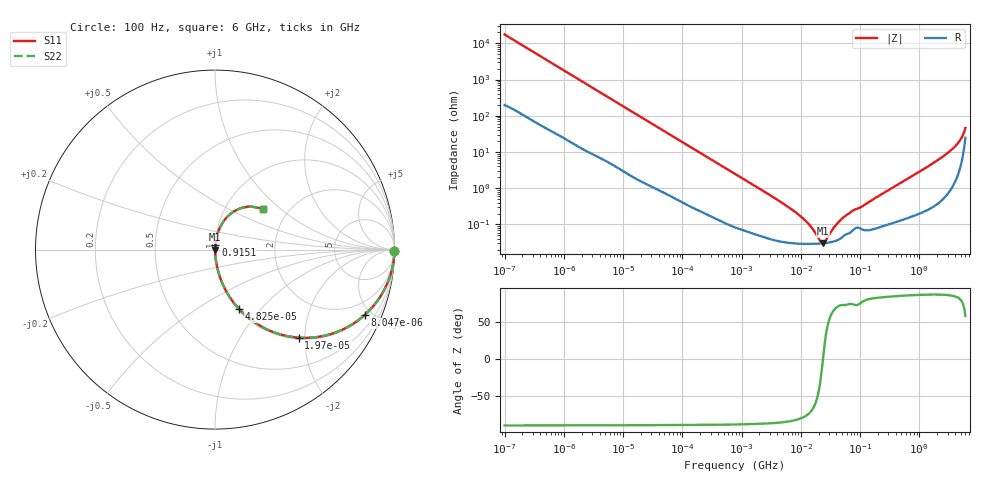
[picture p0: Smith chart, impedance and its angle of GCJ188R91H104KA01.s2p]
!Murata Part Number: GCJ188R91H104KA01
!These Parameters are Measured in Series Mode Connection
!Data Generated on Mar 13, 2026
!  o--ll--o
!Port1  Port2
!  o------o
!Operation Temp=25[degC], DC Bias Voltage=0[V]
!Freq. Start=100[Hz] Stop=6[GHz] 401[Steps]
# Hz S RI R 50
!Freq.(Hz) S11(Real) S11(Imag) S21(Real) S21(Imag) S12(Real) S12(Imag) S22(Real) S22(Imag)
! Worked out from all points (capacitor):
!   401 points, 100 Hz to 6 GHz, reference 50 ohm
!   read as one part in series: C = 90.4 nF near 109 Hz
!   lowest |Z| = 30.3 mohm at 23.28 MHz (marker M1)
!   series resonance near 23.65 MHz, so ESL is about 500 pH
!   S11 on the Smith chart (normalised r, x): 100 Hz: open; 8.047 kHz: 1.07, -4.53; 19.7 kHz: 1.03, -1.87; 48.25 kHz: 1.02, -0.77; 915.1 MHz: 1.00, +0.05; 6 GHz: 1.50, +0.78
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100  0.9999 -0.0057  9.63e-05 0.0057  9.63e-05 0.0057  0.9999 -0.0057
2008  0.9862 -0.1099  0.0138 0.1099  0.0138 0.1099  0.9862 -0.1099
4496  0.9388 -0.232  0.0612 0.232  0.0612 0.232  0.9388 -0.232
8047  0.8331 -0.3649  0.1669 0.3649  0.1669 0.3649  0.8331 -0.3649
19704  0.4663 -0.4906  0.5337 0.4906  0.5337 0.4906  0.4663 -0.4906
40335  0.1791 -0.3739  0.8209 0.3739  0.8209 0.3739  0.1791 -0.3739
48246  0.1341 -0.3309  0.8659 0.3309  0.8659 0.3309  0.1341 -0.3309
161617  0.0161 -0.1145  0.9839 0.1145  0.9839 0.1145  0.0161 -0.1145
774597  0.00145 -0.0248  0.9986 0.0248  0.9986 0.0248  0.00145 -0.0248
6644369  0.000315 -0.00276  0.9997 0.00276  0.9997 0.00276  0.000315 -0.00276
1.087309e7  0.000294 -0.00145  0.9997 0.00145  0.9997 0.00145  0.000294 -0.00145
1.555665e7  0.000291 -0.000728  0.9997 0.000728  0.9997 0.000728  0.000291 -0.000728
2.327686e7  0.000302 -2.68e-05  0.9997 2.68e-05  0.9997 2.68e-05  0.000302 -2.68e-05
2.545746e7  0.000306 0.000125  0.9997 -0.000125  0.9997 -0.000125  0.000306 0.000125
3.64232e7  0.000342 0.000758  0.9997 -0.000758  0.9997 -0.000758  0.000342 0.000758
5.211241e7  0.000475 0.00149  0.9995 -0.00149  0.9995 -0.00149  0.000475 0.00149
3.124326e8  0.0011 0.00908  0.9989 -0.00908  0.9989 -0.00908  0.0011 0.00908
9.150511e8  0.00253 0.0258  0.9975 -0.0258  0.9975 -0.0258  0.00253 0.0258
2.34314e9  0.00917 0.0683  0.9908 -0.0683  0.9908 -0.0683  0.00917 0.0683
4.009986e9  0.0335 0.1346  0.9665 -0.1346  0.9665 -0.1346  0.0335 0.1346
5.016141e9  0.0827 0.1962  0.9173 -0.1962  0.9173 -0.1962  0.0827 0.1962
6e9  0.2699 0.2279  0.7301 -0.2279  0.7301 -0.2279  0.2699 0.2279
